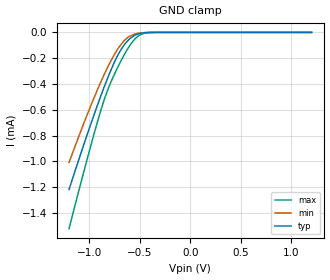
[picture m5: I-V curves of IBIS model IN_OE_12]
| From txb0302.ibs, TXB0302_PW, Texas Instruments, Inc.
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[Model]   IN_OE_12
Model_type  Input
Vinl=0.42
Vinh=0.78
| variable   typ   min   max
C_comp   0.36pF   0.26pF   0.45pF
[Temperature Range]   40   100   -40
| Ambient temperature   25   85   -40
[Voltage range]   1.2   1.1   1.3
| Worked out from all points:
|   GND clamp passes 1 mA (typ) near -1.11 V on its own axis
[GND Clamp]
| IN_OE_12
|   Voltage   I(typ)   I(min)   I(max)
-1.2V     -1.217mA   -1.007mA   -1.52mA
-1.075V   -918.9uA   -747.4uA   -1.142mA
-970mV    -677.3uA   -540uA     -835.8uA
-895mV    -512.5uA   -401.2uA   -629.7uA
-835mV    -387.7uA   -298uA     -483.3uA
-750mV    -228.9uA   -169.9uA   -322.5uA
-680mV    -126.7uA   -87.81uA   -211.2uA
-605mV    -54.11uA   -32.47uA   -109.2uA
-525mV    -14.18uA   -8.274uA   -34.33uA
-465mV    -3.759uA   -2.306uA   -8.986uA
-375mV    -347.7nA   -228.3nA   -560.5nA
1.2V      72.78pA    214.7pA    6.136pA
